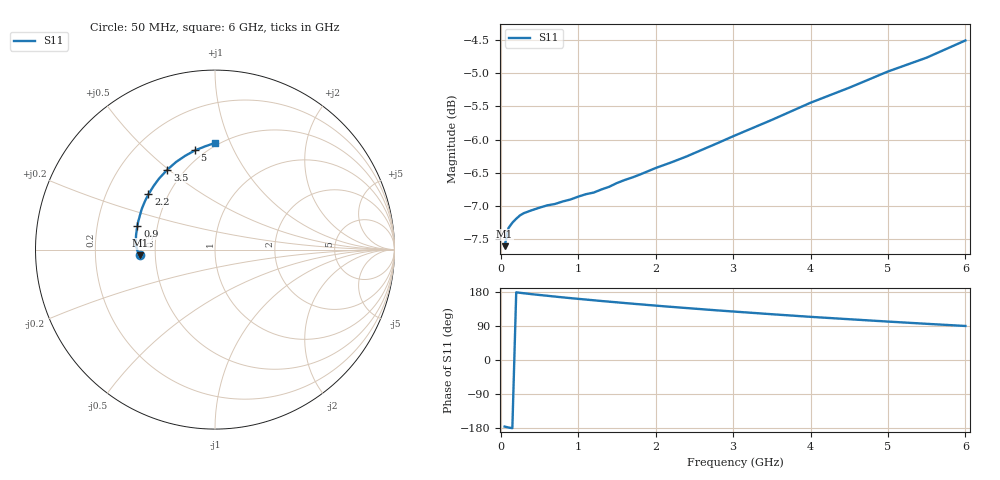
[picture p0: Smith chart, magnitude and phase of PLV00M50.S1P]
! Infineon Technologies  Discrete & RF Semiconductors
! BAR 64-04W /-05W /-06W
! Si PIN Diode in SOT323
! IF = 0.5 mA
! S-Parameters:  October  2008
# GHz  S  MA  R  50
!  f  S11
! GHz  MAG  ANG
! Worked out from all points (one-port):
!   34 points, 50 MHz to 6 GHz, reference 50 ohm
!   lowest |S11| = -7.6 dB at 50 MHz (marker M1), VSWR 2.43, Z = 20.6 - j1.59 ohm
!   |S11| at or under -10 dB: nowhere
!   S11 on the Smith chart (normalised r, x): 50 MHz: 0.41, -0.03; 900 MHz: 0.38, +0.13; 2.2 GHz: 0.39, +0.31; 3.5 GHz: 0.41, +0.49; 5 GHz: 0.44, +0.72; 6 GHz: 0.48, +0.88
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0.05  0.4166 -175.6
0.1  0.4299 -178.2
0.15  0.4339 -179.9
0.2  0.4369 178.6
0.25  0.4395 177.3
0.3  0.4412 176.1
0.4  0.4434 173.7
0.5  0.4453 171.6
0.6  0.4471 169.5
0.8  0.4501 165.3
0.9  0.4517 163.3
1.1  0.4559 159.5
1.2  0.4572 157.6
1.3  0.4596 155.7
1.5  0.4648 152.2
1.6  0.4672 150.4
2  0.477 143.5
2.2  0.4817 140.3
2.4  0.4867 137.1
2.6  0.4924 134.0
2.8  0.4981 130.9
3  0.5041 128.0
3.5  0.5186 120.8
4  0.5343 113.9
4.5  0.5484 107.6
5  0.564 101.4
5.5  0.5777 95.5
6  0.5952 89.8
